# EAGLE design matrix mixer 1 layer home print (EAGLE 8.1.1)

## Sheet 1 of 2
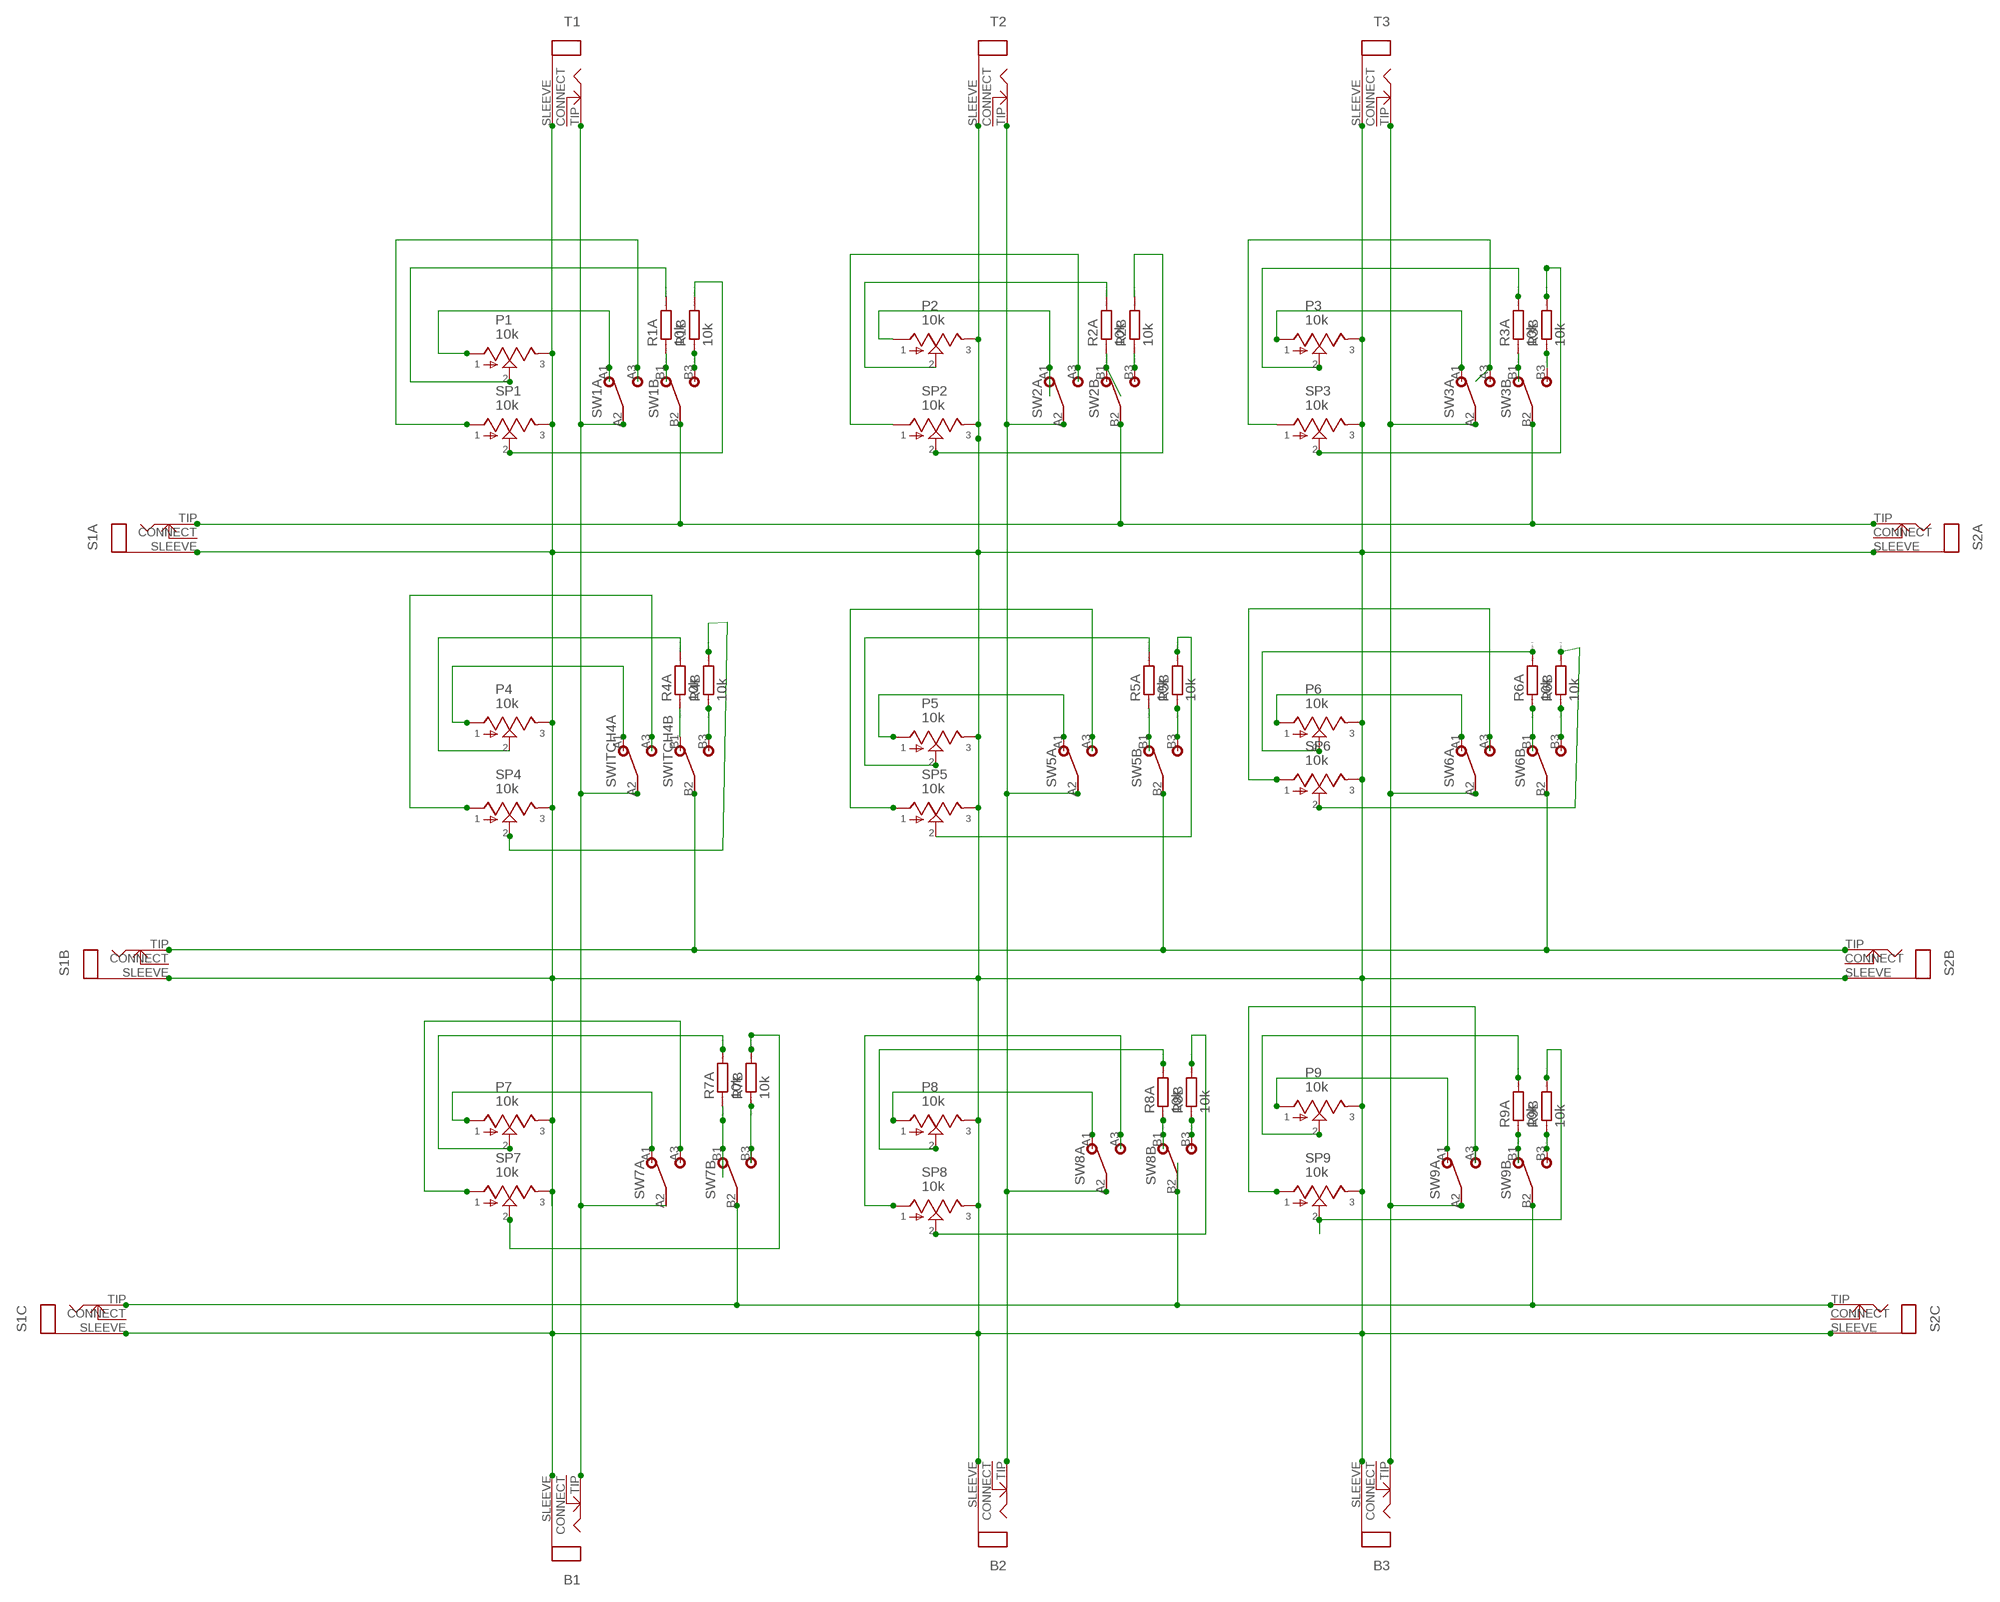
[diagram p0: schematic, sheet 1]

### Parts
B1  CLOSEDMONO  [CLOSED_MONO_JACK]
B2  CLOSEDMONO  [CLOSED_MONO_JACK]
B3  CLOSEDMONO  [CLOSED_MONO_JACK]
P1  10k  POTPCB  [16MM-PCB-MOUNT]
P2  10k  POTPCB  [16MM-PCB-MOUNT]
P3  10k  POTPCB  [16MM-PCB-MOUNT]
P4  10k  POTPCB  [16MM-PCB-MOUNT]
P5  10k  POTPCB  [16MM-PCB-MOUNT]
P6  10k  POTPCB  [16MM-PCB-MOUNT]
P7  10k  POTPCB  [16MM-PCB-MOUNT]
P8  10k  POTPCB  [16MM-PCB-MOUNT]
P9  10k  POTPCB  [16MM-PCB-MOUNT]
R1A  10k  R0204/7  [0204/7]
R1B  10k  R0204/7  [0204/7]
R2A  10k  R0204/7  [0204/7]
R2B  10k  R0204/7  [0204/7]
R3A  10k  R0204/7  [0204/7]
R3B  10k  R0204/7  [0204/7]
R4A  10k  R0204/7  [0204/7]
R4B  10k  R0204/7  [0204/7]
R5A  10k  R0204/7  [0204/7]
R5B  10k  R0204/7  [0204/7]
R6A  10k  R0204/7  [0204/7]
R6B  10k  R0204/7  [0204/7]
R7A  10k  R0204/7  [0204/7]
R7B  10k  R0204/7  [0204/7]
R8A  10k  R0204/7  [0204/7]
R8B  10k  R0204/7  [0204/7]
R9A  10k  R0204/7  [0204/7]
R9B  10k  R0204/7  [0204/7]
S1A  CLOSEDMONO  [CLOSED_MONO_JACK]
S1B  CLOSEDMONO  [CLOSED_MONO_JACK]
S1C  CLOSEDMONO  [CLOSED_MONO_JACK]
S2A  CLOSEDMONO  [CLOSED_MONO_JACK]
S2B  CLOSEDMONO  [CLOSED_MONO_JACK]
S2C  CLOSEDMONO  [CLOSED_MONO_JACK]
SP1  10k  POTPCB  [16MM-PCB-MOUNT]
SP2  10k  POTPCB  [16MM-PCB-MOUNT]
SP3  10k  POTPCB  [16MM-PCB-MOUNT]
SP4  10k  POTPCB  [16MM-PCB-MOUNT]
SP5  10k  POTPCB  [16MM-PCB-MOUNT]
SP6  10k  POTPCB  [16MM-PCB-MOUNT]
SP7  10k  POTPCB  [16MM-PCB-MOUNT]
SP8  10k  POTPCB  [16MM-PCB-MOUNT]
SP9  10k  POTPCB  [16MM-PCB-MOUNT]
SW1  DPDT  [DPDT]
SW2  DPDT  [DPDT]
SW3  DPDT  [DPDT]
SW5  DPDT  [DPDT]
SW6  DPDT  [DPDT]
SW7  DPDT  [DPDT]
SW8  DPDT  [DPDT]
SW9  DPDT  [DPDT]
SWITCH4  DPDT  [DPDT]
T1  CLOSEDMONO  [CLOSED_MONO_JACK]
T2  CLOSEDMONO  [CLOSED_MONO_JACK]
T3  CLOSEDMONO  [CLOSED_MONO_JACK]

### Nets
GND: B1.SLEEVE(RING) B2.SLEEVE(RING) B3.SLEEVE(RING) P1.3 P2.3 P3.3 P4.3 P5.3 P6.3 P7.3 P8.3 P9.3 S1A.SLEEVE(RING) S1B.SLEEVE(RING) S1C.SLEEVE(RING) S2A.SLEEVE(RING) S2B.SLEEVE(RING) S2C.SLEEVE(RING) SP1.3 SP2.3 SP3.3 SP4.3 SP5.3 SP6.3 SP7.3 SP8.3 SP9.3 T1.SLEEVE(RING) T2.SLEEVE(RING) T3.SLEEVE(RING)
N$1: R8A.1 SW8.B1
N$2: P1.1 SW1.A1
N$3: R7A.1 SW7.B1
N$4: R1A.1 SW1.B1
N$5: P7.1 SW7.A1
N$6: P2.2 R2A.2
N$7: P1.2 R1A.2
N$8: R4A.1 SWITCH4.B1
N$9: S1A.TIP S2A.TIP SW1.B2 SW2.B2 SW3.B2
N$10: B1.TIP SW1.A2 SW7.A2 SWITCH4.A2 T1.TIP
N$11: P4.2 R4A.2
N$12: P4.1 SWITCH4.A1
N$13: R7B.1 SW7.B3
N$14: SP4.1 SWITCH4.A3
N$15: R4B.1 SWITCH4.B3
N$16: R4B.2 SP4.2
N$17: S1B.TIP S2B.TIP SW5.B2 SW6.B2 SWITCH4.B2
N$18: SP1.1 SW1.A3
N$19: P7.2 R7A.2
N$20: R7B.2 SP7.2
N$22: SP7.1 SW7.A3
N$23: S1C.TIP S2C.TIP SW7.B2 SW8.B2 SW9.B2
N$24: R2A.1 SW2.B1
N$25: R1B.1 SW1.B3
N$26: SP2.1 SW2.A3
N$27: R1B.2 SP1.2
N$28: P2.1 SW2.A1
N$29: R3A.1 SW3.B1
N$30: B2.TIP SW2.A2 SW5.A2 SW8.A2 T2.TIP
N$31: R2B.2 SP2.2
N$32: SP3.1 SW3.A3
N$33: R2B.1 SW2.B3
N$34: P5.1 SW5.A1
N$35: P5.2 R5A.2
N$36: R5A.1 SW5.B1
N$37: R5B.2 SP5.2
N$38: R5B.1 SW5.B3
N$39: SP5.1 SW5.A3
N$40: P8.1 SW8.A1
N$41: R6A.1 SW6.B1
N$42: R8B.2 SP8.2
N$43: R8B.1 SW8.B3
N$44: P8.2 R8A.2
N$45: P3.1 SW3.A1
N$46: P3.2 R3A.2
N$47: SP6.1 SW6.A3
N$48: B3.TIP SW3.A2 SW6.A2 SW9.A2 T3.TIP
N$49: P6.1 SW6.A1
N$50: P6.2 R6A.2
N$51: SP8.1 SW8.A3
N$52: R6B.1 SW6.B3
N$53: R6B.2 SP6.2
N$54: R9A.1 SW9.B1
N$55: R3B.2 SP3.2
N$56: R3B.1 SW3.B3
N$58: P9.1 SW9.A1
N$59: P9.2 R9A.2
N$60: SP9.1 SW9.A3
N$61: R9B.1 SW9.B3
N$62: R9B.2 SP9.2
Unconnected: B1.CONNECT B2.CONNECT B3.CONNECT S1A.CONNECT S1B.CONNECT S1C.CONNECT S2A.CONNECT S2B.CONNECT S2C.CONNECT T1.CONNECT T2.CONNECT T3.CONNECT

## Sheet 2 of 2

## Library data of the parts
B1-B3 S1A S1B S1C S2A S2B S2C T1-T3 = gm-jacks:CLOSEDMONO: Closed Mono 1/4" Phone Jack
P1-P9 SP1-SP9 = gm-pots:POT: Potentiometers the arrow indicates the clockwise motion of th wiper (lug 2) fully counter clockwise there is no resistance between lugs 1 and 2 fully clockwise the resistance between lugs 1 and 2 is the value of the pot
R1A R1B R2A R2B R3A R3B R4A R4B R5A R5B R6A R6B R7A R7B R8A R8B R9A R9B = eagle-ltspice:R: RESISTOR, European symbol; SPICEMODEL: NONE; SPICEPREFIX: R
SW1-SW3 SW5-SW9 SWITCH4 = gm-switches:DPDT

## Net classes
0 default: width 0.305 mm, drill 0.508 mm, clearance 0.254 mm

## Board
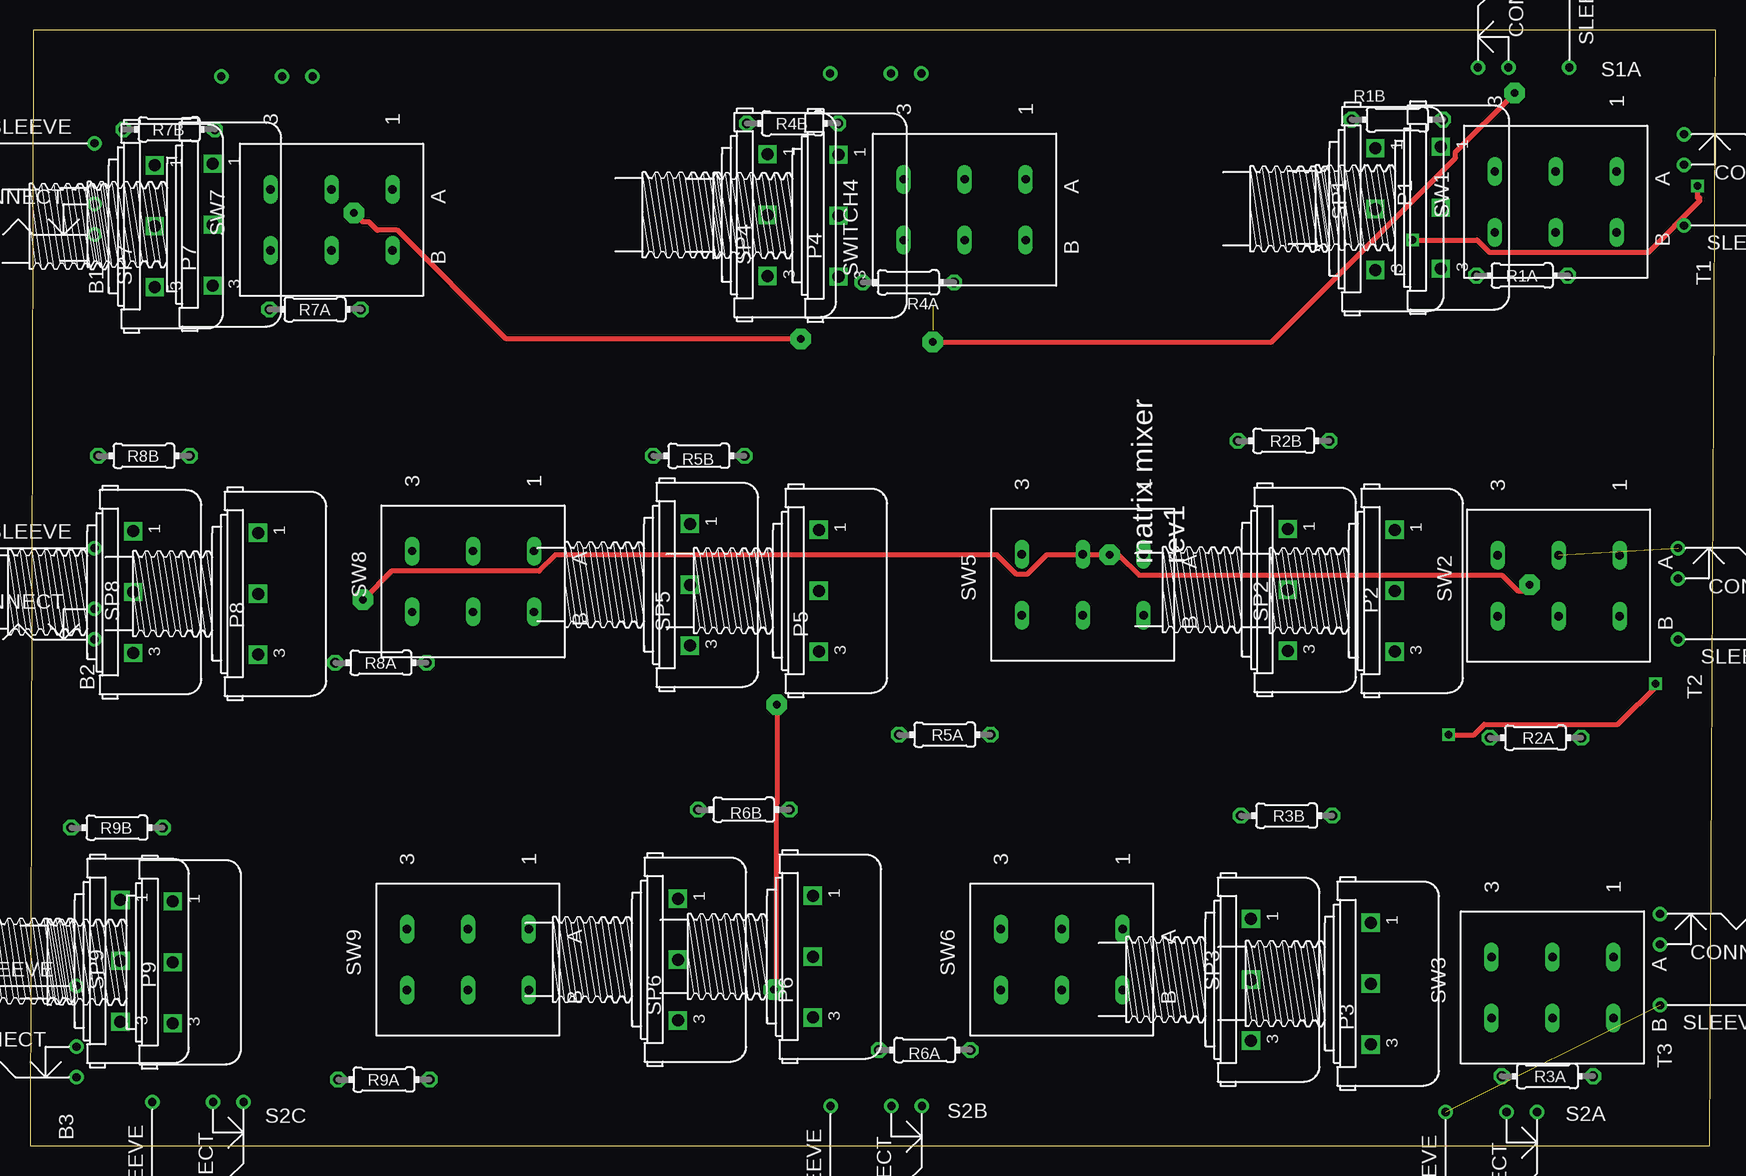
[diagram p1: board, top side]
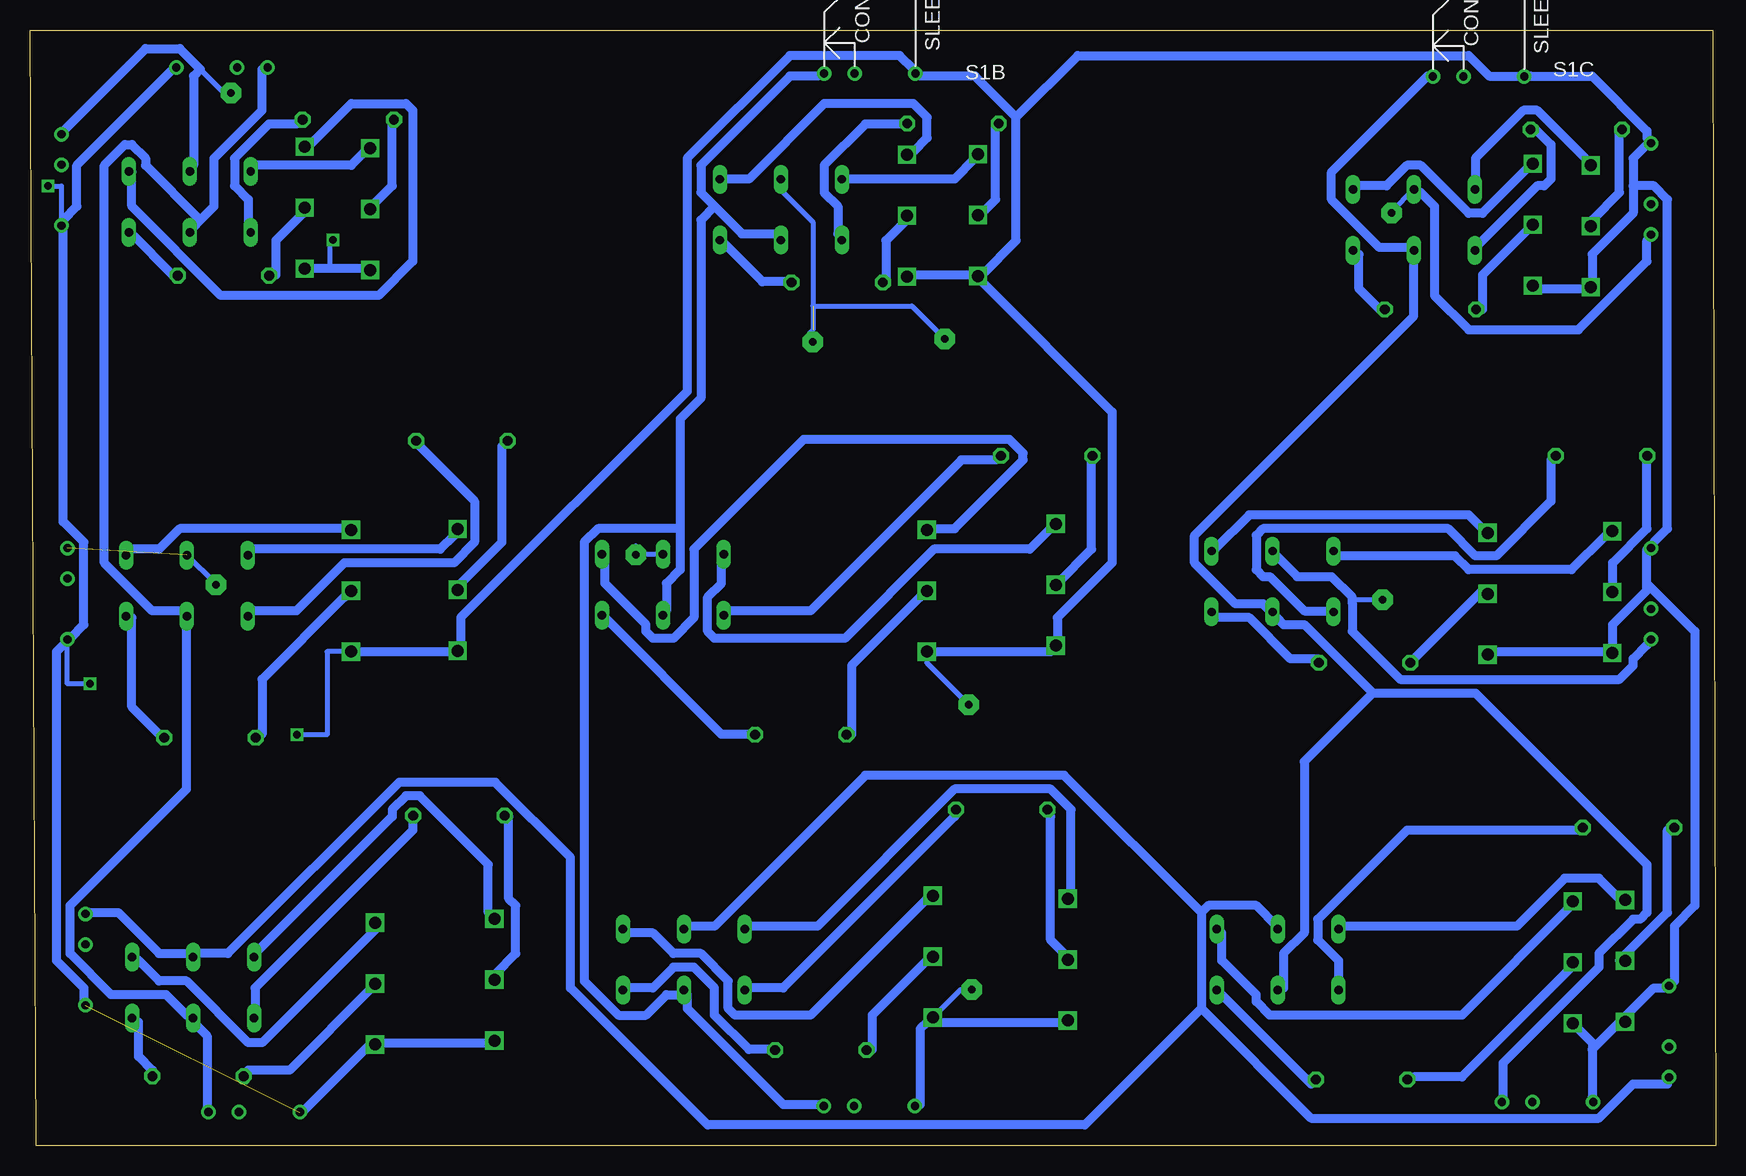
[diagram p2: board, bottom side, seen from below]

Size 140.5 x 93 mm. Coordinates in mm from the lower left corner, seen from the top.
Outline: 0,0 140,0 140.5,93 0.25,93 0,0
Copper layers (1*16): Top 0.035mm / dielectric 1.5mm / Bottom 0.035mm
Design rules "default *": minimum track width 30mil, minimum drill 24mil, track to track 15mil, track to pad 8mil, pad to pad 8mil, via to via 8mil, smd to smd 8mil, copper to edge 40mil, drill to drill 8mil, minimum pad ring 10mil, minimum via ring 8mil, stop-mask expansion 4mil, vias tented up to drill 0mil, thermal gap 10mil

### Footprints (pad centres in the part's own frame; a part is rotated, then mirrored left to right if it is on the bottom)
CLOSED_MONO_JACK = drill 0.7: CONNECT 7.62,-1.27; SLEEVE 7.62,3.81; TIP 7.62,-3.81
16MM-PCB-MOUNT = drill 1 square: 1 5.08,0; 2 0,0; 3 -5.08,0
0204/7 = drill 0.813 octagon: 1 -3.81,0; 2 3.81,0
DPDT = drill 0.7 long: A1 -2.54,5.08; A2 -2.54,0; A3 -2.54,-5.08; B1 2.54,5.08; B2 2.54,0; B3 2.54,-5.08

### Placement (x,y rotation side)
B1  -2.25,79.75 0 top
B2  -2.25,46 0 top
B3  -3.75,9.5 0 top
P1  117.61,78.19 90 top
P2  113.75,46.25 90 top
P3  111.75,13.5 90 top
P4  67.39,77.53 90 top
P5  65.75,46.25 90 top
P6  65.25,15.75 90 top
P7  15.24,76.78 90 top
P8  19,46 90 top
P9  11.89,15.28 90 top
R1A  124.38,72.53 180 top
R1B  113.97,85.53 180 top
R2A  125.5,34 180 top
R2B  104.5,58.75 180 top
R3A  126.49,5.78 180 top
R3B  104.75,27.5 180 top
R4A  73.22,71.96 180 top
R4B  63.56,85.21 180 top
R5A  76.25,34.25 180 top
R5B  55.75,57.5 180 top
R6A  74.58,7.96 180 top
R6B  59.5,28 180 top
R7A  23.76,69.71 180 top
R7B  11.6,84.71 180 top
R8A  29.25,40.25 180 top
R8B  9.5,57.5 180 top
R9A  29.5,5.5 180 top
R9B  7.25,26.5 180 top
S1A  124.5,97.5 270 top
S1B  70.5,97 270 bottom
S1C  19.75,96.75 270 bottom
S2A  121.82,-4.84 90 top
S2B  70.54,-4.34 90 top
S2C  14,-4 90 top
SP1  112.14,78.08 90 top
SP2  104.84,46.33 90 top
SP3  101.79,13.83 90 top
SP4  61.49,77.58 90 top
SP5  55,46.75 90 top
SP6  54,15.5 90 top
SP7  10.39,76.63 90 top
SP8  8.59,46.13 90 top
SP9  7.54,15.38 90 top
SW1  127.18,78.68 270 top
SW2  127.42,46.68 270 top
SW3  126.91,13.18 270 top
SW5  87.75,46.75 270 top
SW6  86,15.5 270 top
SW7  25.13,77.18 270 top
SW8  36.93,47.02 270 top
SW9  36.5,15.5 270 top
SWITCH4  77.91,78.02 270 top
T1  145.5,80.5 180 top
T2  145,46 180 top
T3  143.5,15.5 180 top

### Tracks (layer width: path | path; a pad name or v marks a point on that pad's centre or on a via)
GND  (via drill 0.6, 0.6 pad 1.68)  (1 unrouted)
  Top 0.406: v62.25,36.75 62.25,28.52 62.19,28.46 62.19,13.69 62,13.5 v62,13 | v118.25,34.25 120.36,34.25 121.23,35.12 132.37,35.12 135.75,38.5 v135.5,38.5 | v115.25,75.5 120.64,75.5 121.66,74.47 134.93,74.47 139.2,78.75 139.21,79 139,79 v139,80
  Bottom 0.406: P5.3 65.75,40.25 v62.25,36.75 | v62,13 62.92,13 P6.3 | P2.3 115.75,41.17 115.75,34.25 v118.25,34.25 | v135.5,38.5 137.38,38.5 T2.SLEEVE | P1.3 115.5,73.11 115.5,75.5 v115.25,75.5 | v139,80 137.88,80 T1.SLEEVE
  Bottom 0.762: P7.3 14.86,71.44 10.86,71.44 SP7.3 10.29,72.01 10.29,74.3 6.86,77.72 6.86,80.01 | 6.86,80.01 6.86,82.3 5.71,83.44 B1.SLEEVE 5.71,84.01 5.71,84.58 10.29,89.15 15.43,89.15 S1C.SLEEVE 16,89.15 18.86,89.15 20.57,90.87 53.15,90.87 58.29,85.72 | 10.29,8 10.29,8.57 11.43,9.72 P9.3 | 10.29,8 10.29,4 S2C.SLEEVE | 10.29,8 8,10.29 SP9.3 7.43,10.86 5.14,13.14 4,13.14 B3.SLEEVE 3.43,13.72 3.43,18.29 1.71,20 1.71,42.86 5.71,46.86 | 5.71,46.86 5.71,46.29 8.57,43.43 8.57,41.15 SP8.3 9.14,41.15 18.86,41.15 P8.3 | 5.71,46.86 5.71,49.72 B2.SLEEVE 5.14,50.29 4,51.44 4,78.87 5.14,80.01 6.86,80.01 | P5.3 65.72,41.15 55.44,41.15 SP5.3 54.86,41.72 54.86,44.01 50.29,48.58 50.29,61.15 61.15,72.01 SP4.3 | P2.3 113.73,41.15 105.16,41.15 SP2.3 104.58,41.72 104.58,44.01 85.72,62.87 85.72,82.3 77.15,90.87 68.01,90.87 66.86,89.72 S1B.SLEEVE 66.29,89.15 61.72,89.15 58.29,85.72 | 58.29,85.72 58.29,75.44 61.15,72.58 SP4.3 | P4.3 66.86,72.58 61.72,72.58 SP4.3 | S2B.SLEEVE 66.29,3.43 66.29,9.72 65.72,10.29 P6.3 65.15,10.29 54.29,10.29 SP6.3 | S2A.SLEEVE 117.73,2.86 112.01,8.57 P3.3 111.44,8.57 102.3,8.57 SP3.3 | SP1.3 112.58,73.15 117.16,73.15 P1.3 | S1A.SLEEVE 128.59,89.72 136.59,81.72 136.59,78.3 137.73,77.15 T1.SLEEVE 137.73,76.58 137.73,52.01 136.02,50.29 136.02,43.43 137.16,42.29 T2.SLEEVE 137.73,41.72 138.3,41.15 138.3,15.43 136.02,13.14 136.02,12 T3.SLEEVE
N$1
  Bottom 0.762: SW8.B1 41.72,44.01 38.86,44.01 35.43,40.58 33.15,40.58 R8A.1
N$2
  Bottom 0.762: SW1.A1 132.02,81.15 132.02,78.3 124.59,70.87 111.44,70.87 108.58,73.72 108.58,86.3 109.16,86.87 113.73,86.87 117.16,83.44 P1.1
N$3
  Bottom 0.762: SW7.B1 29.72,74.3 29.72,71.44 28,69.72 R7A.1
N$4
  Bottom 0.762: SW1.B1 132.02,76.01 128.59,72.58 R1A.1
N$5
  Bottom 0.762: SW7.A1 29.72,80.01 27.43,80.01 25.72,81.72 24.57,81.72 20.57,77.72 19.43,77.72 15.43,81.72 P7.1
N$6
  Bottom 0.762: R2A.2 121.16,34.29 121.16,38.86 114.3,45.72 P2.2
N$7
  Bottom 0.762: R1A.2 120.02,72.58 120.02,75.44 117.73,77.72 P1.2
N$8
  Bottom 0.762: SWITCH4.B1 82.87,75.44 79.44,72.01 77.15,72.01 R4A.1
N$9
  Bottom 0.762: 126.3,77.15 126.87,76.58 SW1.B2 | 126.3,77.15 125.16,78.3 125.16,82.3 121.16,86.3 121.16,89.72 S1A.TIP | S2A.TIP 125.73,2.86 125.73,9.14 126.87,10.29 SW3.B2 127.44,10.86 129.16,12.57 133.73,12.57 137.16,16 137.16,20 127.44,29.72 127.44,44.01 SW2.B2 127.44,44.58 130.3,44.58 134.3,48.58 134.3,81.72 132.59,83.44 132.02,83.44 130.87,82.3 130.87,81.72 126.3,77.15
N$10  (via drill 0.6 pad 1.68)  (1 unrouted)
  Top 0.406: v123.75,87.75 118.82,82.82 118.82,82.33 103.5,67 v75.25,67 | v123.75,87.75 124,88 v123.75,87.75 | v64.25,67.25 39.7,67.25 30.65,76.31 28.95,76.31 28.25,77 27.75,77 v27,77.75
  Bottom 0.406: SWITCH4.A2 77.91,79.66 75.25,77 75.25,68 75.5,67.75 75.5,67.25 v75.25,67 | v123.75,87.75 124.33,87.75 126.3,89.72 | v64.25,67.25 67,70 75.25,70 | v27,77.75 27,77.85 SW7.A2
  Bottom 0.762: SW1.A2 126.87,81.72 126.87,89.15 126.3,89.72 128.02,91.44 130.87,91.44 137.73,84.58 T1.TIP | B1.TIP 5.71,75.44 5.71,73.72 11.43,68.01 20.57,68.01 23.43,70.87 23.43,78.3 24.57,79.44 SW7.A2
N$11
  Bottom 0.762: R4A.2 69.15,72.01 69.15,75.44 67.44,77.15 P4.2
N$12
  Bottom 0.762: SWITCH4.A1 82.87,80.58 80.58,80.58 74.3,86.87 66.86,86.87 65.72,85.72 65.72,84.01 66.86,82.87 P4.1
N$13
  Bottom 0.762: SW7.B3 20,74.87 14.86,80.01 14.29,80.01 13.72,80.58 13.72,83.44 14.86,84.58 R7B.1
N$14
  Bottom 0.762: SWITCH4.A3 72.58,80.58 63.44,80.58 61.72,82.3 SP4.1
N$15
  Bottom 0.762: SWITCH4.B3 73.15,76.01 73.15,78.3 74.3,79.44 74.3,81.72 70.87,85.15 67.44,85.15 R4B.1
N$16
  Bottom 0.762: R4B.2 60.01,85.15 60.01,78.87 61.15,77.72 SP4.2
N$17
  Bottom 0.762: S2B.TIP 74.87,3.43 77.72,3.43 85.72,11.43 85.72,12.57 SW6.B2 86.3,12.57 87.44,12.57 89.15,10.86 91.44,10.86 94.3,13.72 94.3,50.29 93.15,51.44 86.3,51.44 | 83.44,78.3 84.58,79.44 84.58,81.72 77.15,89.15 74.87,89.15 S1B.TIP | 83.44,78.3 81.15,76.01 78.3,76.01 SWITCH4.B2 | 86.3,51.44 86.3,60.58 84.58,62.29 84.58,77.15 83.44,78.3 | 86.3,51.44 86.3,48.01 87.44,46.86 87.44,44.58 SW5.B2
N$18
  Bottom 0.762: SW1.A3 121.73,81.72 113.73,81.72 112.58,82.87 SP1.1
N$19
  Bottom 0.762: R7A.2 19.43,69.72 19.43,72.58 15.43,76.58 P7.2
N$20
  Bottom 0.762: R7B.2 8,84.58 8,79.44 10.29,77.15 SP7.2
N$22
  Bottom 0.762: SW7.A3 20,80.01 20,82.3 16,86.3 14.86,86.3 10.29,81.72 SP7.1
N$23
  Bottom 0.762: S1C.TIP 24,89.15 32,81.15 32,78.87 28,74.87 25.15,74.87 SW7.B2 25.15,74.3 25.15,69.15 43.43,50.86 43.43,48.58 40.01,45.15 37.72,45.15 37.15,44.58 SW8.B2 36.58,44.01 36.01,43.43 34.29,43.43 28.57,37.72 | 28.57,37.72 20,37.72 5.71,23.43 5.71,19.43 6.29,18.86 6.86,18.86 9.72,16 9.72,14.86 17.72,6.86 17.72,4 S2C.TIP | 28.57,37.72 34.29,32 34.29,17.72 36.01,16 36.01,13.14 SW9.B2
N$24
  Bottom 0.762: SW2.B1 132.02,44.01 132.02,36.58 129.73,34.29 R2A.1
N$25
  Bottom 0.762: SW1.B3 122.3,76.58 122.3,78.87 123.44,80.01 123.44,82.3 120.59,85.15 118.3,85.15 R1B.1
N$26
  Bottom 0.762: SW2.A3 122.3,49.72 106.3,49.72 105.16,50.86 SP2.1
N$27
  Bottom 0.762: R1B.2 110.3,85.15 110.3,80.01 112.01,78.3 SP1.2
N$28
  Bottom 0.762: SW2.A1 132.02,49.72 129.73,49.72 128.02,51.44 114.3,51.44 P2.1
N$29
  Bottom 0.762: SW3.B1 131.44,10.29 131.44,7.43 130.3,6.29 R3A.1
N$30  (via drill 0.6 pad 1.68)  (1 unrouted)
  Top 0.406: v125,46.75 124.5,46.25 124,46.25 122.69,47.55 92.46,47.55 90.77,49.25 v90,49.25 84.73,49.25 83.11,47.62 82.23,47.62 80.61,49.25 43.8,49.25 42.45,47.9 30.14,47.9 v27.75,45.5 | v27.75,45.5 27.5,45.25 v27.75,45.5
  Bottom 0.406: SW5.A2 89.96,49.29 v90,49.25 90,50 | v125,46.75 125,46.8 SW2.A2 | v27.75,45.5 30.04,45.5 30.29,45.25
  Bottom 0.762: B2.TIP 5.71,41.72 6.86,40.58 6.86,40.01 8,38.86 26.29,38.86 30.29,42.86 30.29,45.25 30.29,45.72 32,47.43 34.86,47.43 36.58,49.15 SW8.A2
N$31
  Bottom 0.762: R2B.2 101.16,58.29 101.16,50.29 104.58,46.86 SP2.2
N$32
  Bottom 0.762: SW3.A3 121.73,16 110.3,27.43 110.3,28 109.16,29.15 108.01,29.15 102.3,23.43 102.3,19.43 SP3.1
N$33
  Bottom 0.762: SW2.B3 122.3,44.58 118.3,44.58 114.3,48.58 105.16,48.58 103.44,50.29 103.44,53.72 108.01,58.29 R2B.1
N$34
  Bottom 0.762: SW5.A1 92.58,49.15 92.58,46.86 89.15,43.43 89.15,42.86 88.58,42.29 86.87,42.29 85.15,44.01 85.15,49.72 76.01,58.86 58.86,58.86 57.72,57.72 57.72,57.15 63.44,51.44 65.72,51.44 P5.1
N$35
  Bottom 0.762: R5A.2 72.01,34.29 72.01,40.01 66.29,45.72 P5.2
N$36
  Bottom 0.762: SW5.B1 92.58,44.01 82.87,34.29 80.58,34.29 R5A.1
N$37
  Bottom 0.762: R5B.2 52.01,57.15 52.01,49.72 54.86,46.86 SP5.2
N$38
  Bottom 0.762: SW5.B3 82.3,44.58 75.44,44.58 62.87,57.15 60.01,57.15 R5B.1
N$39
  Bottom 0.762: SW5.A3 82.87,49.15 82.87,46.86 84.01,45.72 84.01,42.86 83.44,42.29 72.58,42.29 65.15,49.72 57.15,49.72 55.44,51.44 SP5.1
N$40
  Bottom 0.762: SW8.A1 41.72,49.72 38.86,52.58 20.57,52.58 19.43,51.44 P8.1
N$41
  Bottom 0.762: SW6.B1 90.87,13.14 88.58,13.14 86.87,14.86 85.15,14.86 83.44,13.14 83.44,10.86 80.58,8 78.87,8 R6A.1
N$42
  Bottom 0.762: R8B.2 5.71,57.15 5.71,51.44 8.57,48.58 8.57,46.29 SP8.2
N$43
  Bottom 0.762: SW8.B3 32,44.58 34.29,44.58 37.15,47.43 37.72,47.43 38.29,48.01 38.29,50.86 37.72,51.44 22.29,51.44 20,49.15 18.29,49.15 13.72,53.72 13.72,57.15 R8B.1
N$44
  Bottom 0.762: R8A.2 25.15,40.58 19.43,46.29 P8.2
N$45
  Bottom 0.762: SW3.A1 131.44,15.43 129.73,13.72 127.44,13.72 122.3,8.57 121.16,8.57 111.44,18.29 P3.1
N$46
  Bottom 0.762: R3A.2 122.3,6.29 118.87,6.29 112.01,13.14 P3.2
N$47
  Bottom 0.762: SW6.A3 80.58,18.29 74.87,18.29 63.44,29.72 55.44,29.72 53.72,28 53.72,21.14 SP6.1
N$48
  Bottom 0.762: T3.TIP 135.45,19.43 133.16,19.43 129.73,16 127.44,16 SW3.A2 126.87,16 124.02,16 109.73,30.29 101.73,30.29 95.44,24 95.44,13.14 84.01,1.71 52.58,1.71 42.86,11.43 | 42.86,11.43 33.72,2.29 9.72,2.29 6.86,5.14 4,5.14 B3.TIP | 42.86,19.43 42.86,11.43 | 42.86,19.43 42.29,20 38.29,20 36.58,18.29 SW9.A2 | 42.86,19.43 54.29,30.86 70.87,30.86 83.44,18.29 85.72,18.29 SW6.A2
N$49
  Bottom 0.762: SW6.A1 90.87,17.72 88.58,17.72 86.87,16 84.58,16 82.3,13.72 82.3,11.43 81.72,10.86 75.44,10.86 65.72,20.57 P6.1
N$50
  Bottom 0.762: R6A.2 70.29,8 70.29,10.86 65.72,15.43 P6.2
N$51
  Bottom 0.762: SW8.A3 31.43,49.15 21.72,49.15 20.57,48.01 12,48.01 9.14,50.86 SP8.1
N$52
  Bottom 0.762: SW6.B3 80.58,13.14 77.72,13.14 63.44,27.43 R6B.1
N$53
  Bottom 0.762: R6B.2 55.44,27.43 55.44,17.14 54.29,16 SP6.2
N$54
  Bottom 0.762: SW9.B1 41.15,12.57 33.72,5.14 R9A.1
N$55
  Bottom 0.762: R3B.2 100.58,27.43 100.58,20.57 100.01,20 100.01,16 101.73,14.29 SP3.2
N$56
  Bottom 0.762: SW3.B3 121.73,10.86 121.73,13.14 108.58,26.29 108.58,27.43 R3B.1
N$58
  Bottom 0.762: SW9.A1 41.15,17.72 41.15,15.43 38.29,12.57 38.29,12 37.15,10.86 21.14,10.86 12,20 P9.1
N$59
  Bottom 0.762: R9A.2 25.15,5.71 21.14,5.71 12,14.86 P9.2
N$60
  Bottom 0.762: SW9.A3 30.86,18.29 16.57,18.29 12.57,22.29 9.72,22.29 8,20.57 SP9.1
N$61
  Bottom 0.762: SW9.B3 31.43,13.14 31.43,15.43 33.15,17.14 33.15,18.86 25.72,26.29 11.43,26.29 R9B.1
N$62
  Bottom 0.762: R9B.2 4,26.29 4,19.43 8,15.43 SP9.2

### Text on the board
tPlace: matrix mixer / rev1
